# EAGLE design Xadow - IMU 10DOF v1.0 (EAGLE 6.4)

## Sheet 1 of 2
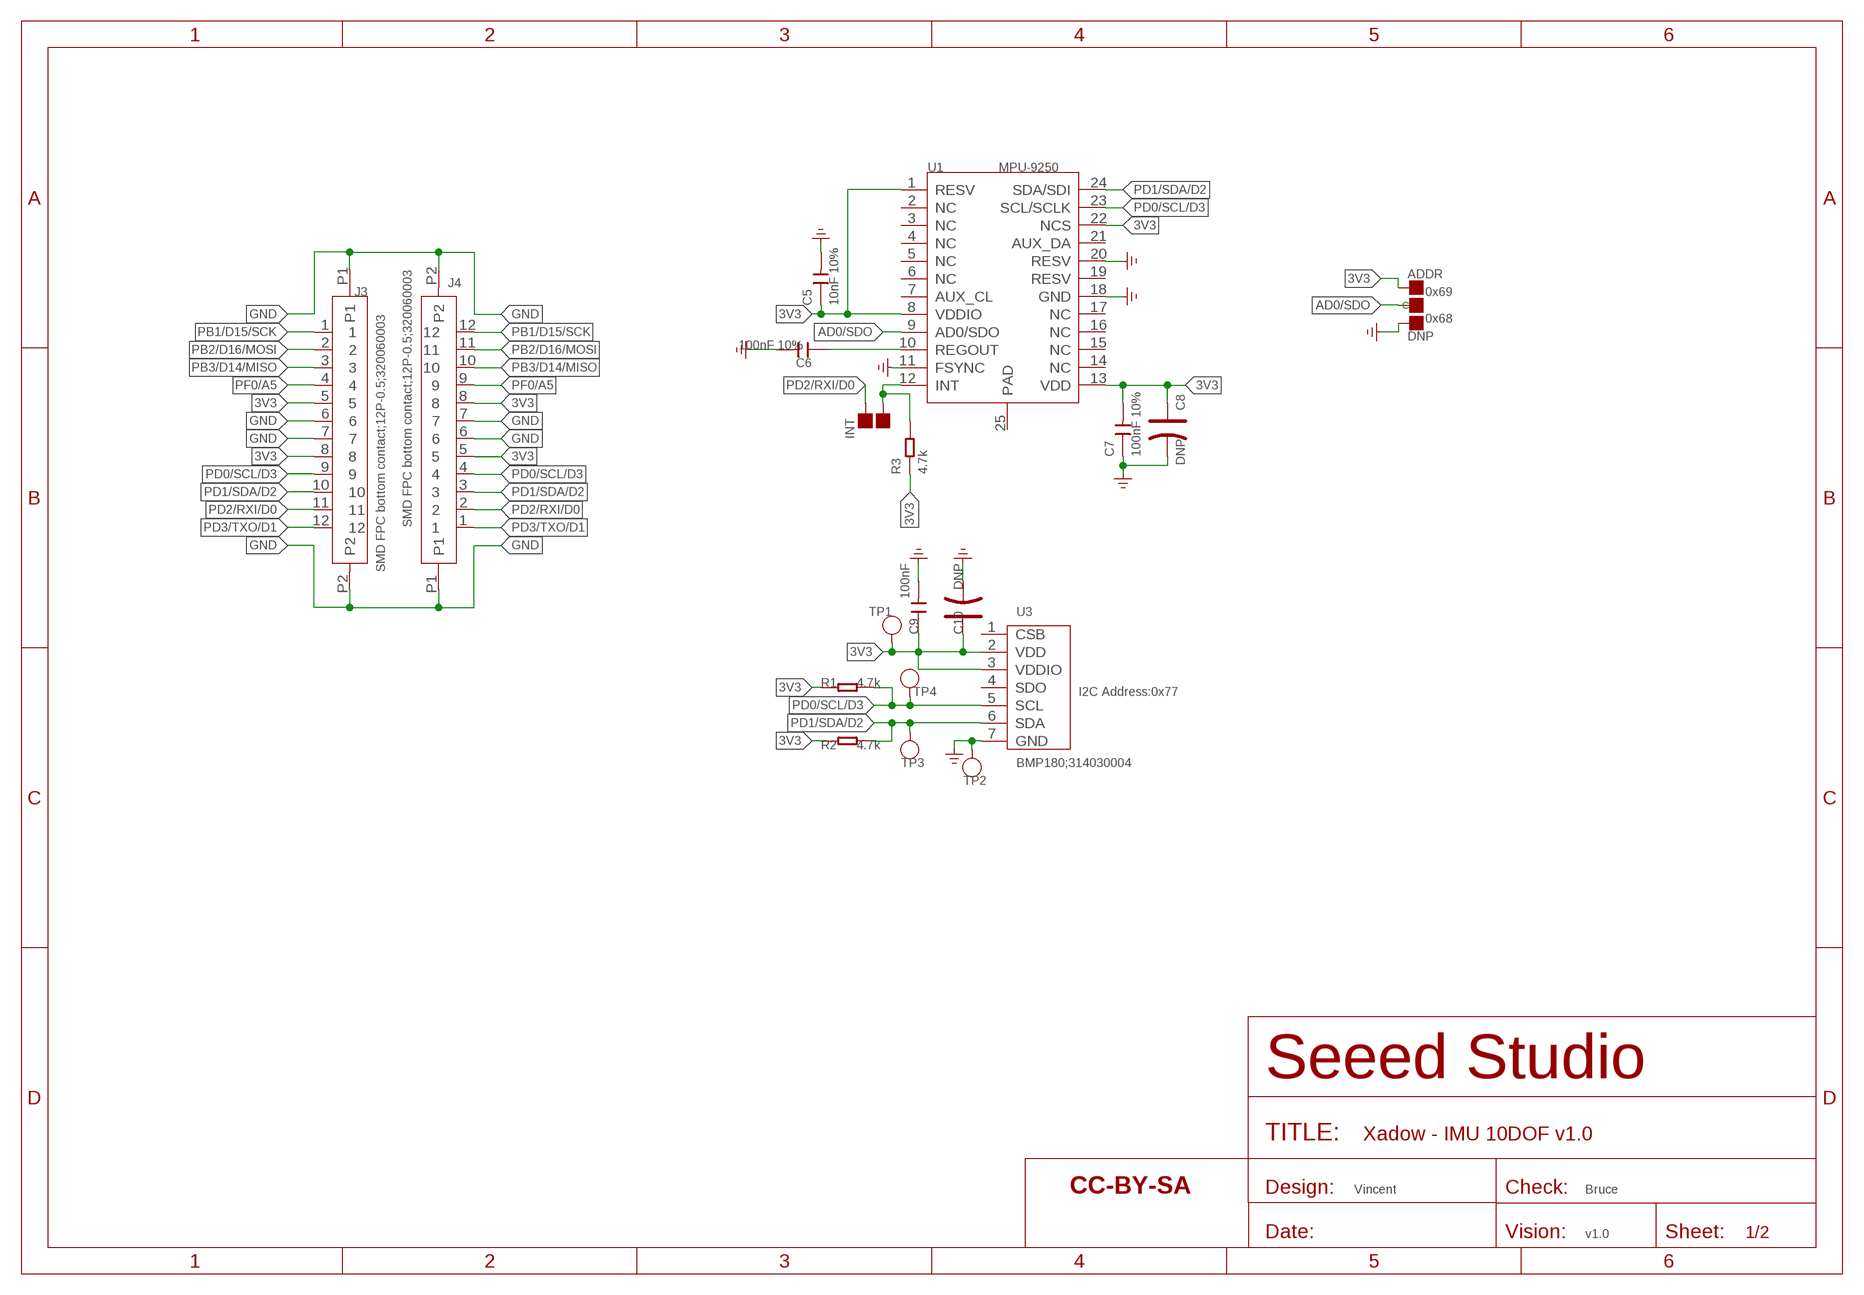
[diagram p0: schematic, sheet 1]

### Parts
ADDR  DNP  PAD-JUMPER-3P-40*40  [3P-SMD-L4.1*W1.5MM]
C5  10nF 10%  CAP-0603  [C0603]
C6  100nF 10%  CAP-0603  [C0603]
C7  100nF 10%  CAP-0603  [C0603]
C8  DNP  CAP-POLAR-AVX-A  [AVX-A]
C9  100nF  CAP-0603  [C0603]
C10  DNP  CAP-POLAR-AVX-A  [AVX-A]
INT  PAD-JUMPER-2P  [2P-SMD-L1.78*W1.27MM]
J3  SMD FPC bottom contact;12P-0.5;320060003  FPC-CONNECTOR-12P-FH12-12S-0.5SH  [12P-0.5]
J4  SMD FPC bottom contact;12P-0.5;320060003  FPC-CONNECTOR-12P-FH12-12S-0.5SH  [12P-0.5]
R1  4.7k  RES-0603  [R0603]
R2  4.7k  RES-0603  [R0603]
R3  4.7k  RES-0603  [R0603]
TP1  PAD-TEST-POINT'4545'  [TP-D45MIL]
TP2  PAD-TEST-POINT'4545'  [TP-D45MIL]
TP3  PAD-TEST-POINT'4545'  [TP-D45MIL]
TP4  PAD-TEST-POINT'4545'  [TP-D45MIL]
U1  MPU-9250  [LEAD-QFN24]
U3  BMP180;314030004  BMP180  [LGA-7]
U$1  SEEEDSTUDIO-OPEN-SCH-FRAME  [SEEEDSTUDIO-PCB-FRAME]

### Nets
3V3: ADDR.00(L) C5.1 C7.2 C8.+ C9.1 C10.+ J3.5 J3.8 J4.5 J4.8 R1.1 R2.1 R3.1 TP1.T U1.1(RESV) U1.8(VDDIO) U1.13(VDD) U1.22(NCS) U3.2(VDD) U3.3(VDDIO)
AD0/SDO: ADDR.MM(C) U1.9(AD0/SDO)
GND: ADDR.11(R) C5.2 C6.2 C7.1 C8.- C9.2 C10.- J3.6 J3.7 J3.P1 J3.P2 J4.6 J4.7 J4.P1 J4.P2 TP2.T U1.11(FSYNC) U1.18(GND) U1.20(RESV) U3.7(GND) ; supply symbol labelled GND_POWER
N$3: C6.1 U1.10(REGOUT)
N$4: INT.1 R3.2 U1.12(INT)
PB1/D15/SCK: J3.1 J4.12
PB2/D16/MOSI: J3.2 J4.11
PB3/D14/MISO: J3.3 J4.10
PD0/SCL/D3: J3.9 J4.4 R1.2 TP4.T U1.23(SCL/SCLK) U3.5(SCL)
PD1/SDA/D2: J3.10 J4.3 R2.2 TP3.T U1.24(SDA/SDI) U3.6(SDA)
PD2/RXI/D0: INT.2 J3.11 J4.2
PD3/TXO/D1: J3.12 J4.1
PF0/A5: J3.4 J4.9
Unconnected: U1.2(NC) U1.3(NC) U1.4(NC) U1.5(NC) U1.6(NC) U1.7(AUX_CL) U1.14(NC) U1.15(NC) U1.16(NC) U1.17(NC) U1.19(RESV) U1.21(AUX_DA) U1.25(PAD) U3.1(CSB) U3.4(SDO)

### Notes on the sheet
- 0x69
- 0x68
- I2C Address:0x77
- Vincent | Bruce
- v1.0

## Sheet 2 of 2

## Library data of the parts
ADDR = Discrete-new:PAD-JUMPER-3P; PARTNO: DNP
C5-C7 C9 = Discrete-new:CAP: Ceramic Capacitors
C8 C10 = Discrete-new:CAP-POLAR: Electrolytic Capacitors,Tantalum Capacitors and Super Capacitors
INT = Discrete-new:PAD-JUMPER-2P; PARTNO: DNP
J3 J4 = Connector-new:FPC-CONNECTOR-12P: 320060003
R1-R3 = Discrete-new:RES
TP1-TP4 = Discrete-new:PAD-TEST-POINT; PARTNO: DNP
U1 = template:MPU-9250
U3 = template:BMP180: Digital pressure sensor
U$1 = moudle-new:SEEEDSTUDIO-OPEN-SCH-FRAME

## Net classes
0 default: width 0.152 mm, drill 0.305 mm, clearance 0.152 mm

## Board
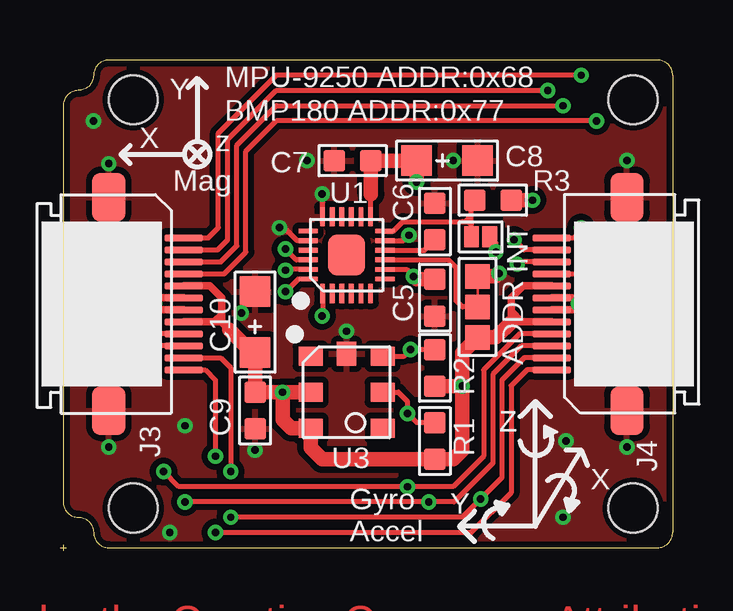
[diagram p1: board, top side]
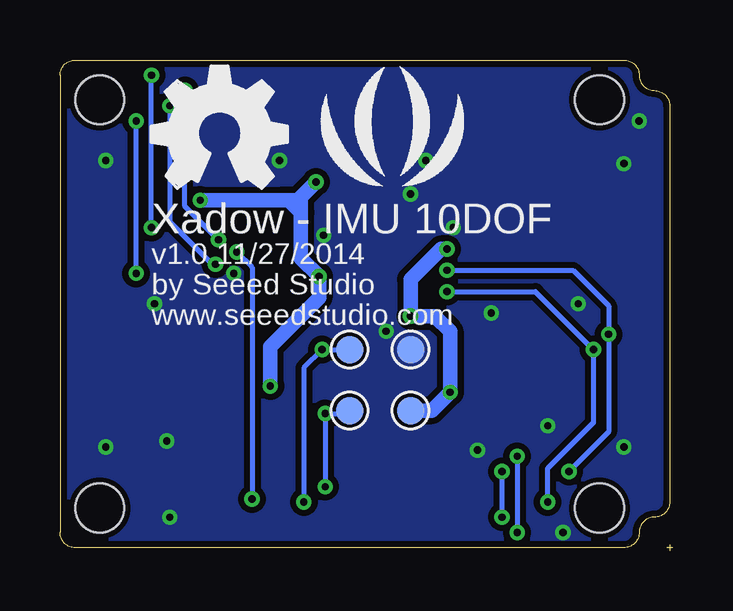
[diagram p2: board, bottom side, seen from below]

Size 25.53 x 20.45 mm. Coordinates in mm from the lower left corner, seen from the top.
Copper layers (1*16): Top 0.035mm / dielectric 1.5mm / Bottom 0.035mm
Design rules "SeeedStudio_2layer_DRU_no_angle_20140221 *": minimum track width 6mil, minimum drill 12mil, track to track 6mil, track to pad 6mil, pad to pad 6mil, via to via 6mil, smd to smd 0mil, copper to edge 10mil, drill to drill 10mil, minimum pad ring 10mil, minimum via ring 6mil, stop-mask expansion 2mil, vias tented up to drill 25mil, thermal gap 10mil

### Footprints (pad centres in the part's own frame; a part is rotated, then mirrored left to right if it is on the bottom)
3P-SMD-L4.1*W1.5MM = smd 1.016 x 1.016: 00 -1.27,0; 11 1.27,0; MM 0,0
C0603 = smd 0.889 x 0.889: 1 0,0.762; 2 0,-0.762
AVX-A = smd 1.27 x 1.27: + -1.27,0; - 1.27,0
2P-SMD-L1.78*W1.27MM = smd 0.889 x 0.61: 1 0,0.381; 2 0,-0.381
12P-0.5 = smd 0.3 x 1.6: 1 -2.75,3.127; 2 -2.25,3.127; 3 -1.75,3.127; 4 -1.25,3.127; 5 -0.75,3.127; 6 -0.25,3.127; 7 0.25,3.127; 8 0.75,3.127; 9 1.25,3.127; 10 1.75,3.127; 11 2.25,3.127; 12 2.75,3.127 | smd 2.032 x 1.397: P1 -4.445,0; P2 4.445,0
R0603 = smd 0.889 x 0.889: 1 0,0.762; 2 0,-0.762
TP-D45MIL = smd 1.143 x 1.143: T 0,0
LEAD-QFN24 = smd 0.8 x 0.2: 1 -1.6,1; 2 -1.6,0.6; 3 -1.6,0.2; 4 -1.6,-0.2; 5 -1.6,-0.6; 6 -1.6,-1; 13 1.6,-1; 14 1.6,-0.6; 15 1.6,-0.2; 16 1.6,0.2; 17 1.6,0.6; 18 1.6,1 | smd 0.2 x 0.8: 7 -1,-1.6; 8 -0.6,-1.6; 9 -0.2,-1.6; 10 0.2,-1.6; 11 0.6,-1.6; 12 1,-1.6; 19 1,1.6; 20 0.6,1.6; 21 0.2,1.6; 22 -0.2,1.6; 23 -0.6,1.6; 24 -1,1.6 | smd 1.7 x 1.54: 25 0,0
LGA-7 = smd 0.8 x 1: 1 1.5,1.5; 2 0,1.5; 3 -1.5,1.5; 4 -1.5,-1.5; 5 0,-1.5; 6 1.5,-1.5 | smd 1 x 0.8: 7 1.6,0
XADOW-DRILL-DIM-25*20MM = hole 2.032: -9.779,-8.509; -9.779,8.509; 11.049,8.509; 11.049,-8.509

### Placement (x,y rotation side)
ADDR  17.4,10.16 90 top
C5  15.62,10.54 0 top
C6  15.62,13.72 180 top
C7  12.19,16.26 90 top
C8  16.13,16.26 0 top
C9  8.13,5.84 0 top
C10  8.13,9.53 90 top
INT  17.53,13.08 90 top
J3  2.03,10.29 270 top
J4  23.62,10.29 90 top
R1  15.62,4.57 180 top
R2  15.62,7.62 180 top
R3  18.03,14.61 270 top
TP1  10.92,5.84 90 bottom
TP2  10.92,8.38 90 bottom
TP3  13.46,8.38 90 bottom
TP4  13.46,5.84 90 bottom
U1  11.94,12.32 90 top
U3  11.94,6.6 90 top
U$1  not placed on the board
U$2  [OSHW_FILLX200_NOTEXT]  21.72,15.11 0 bottom
U$3  [SEEED-SILK-280*268MIL]  11.68,16.89 0 bottom
U$4  [XADOW-DRILL-DIM-25*20MM]  12.83,10.29 0 top
U$15  [XADOW-DRILL-DIM-25*20MM]  12.83,10.29 0 top

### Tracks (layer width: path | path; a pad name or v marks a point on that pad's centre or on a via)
3V3  (via drill 0.3 pad 0.64)
  Top 0.203: U1.13 12.94,14.84 12.95,14.86 | U1.8 14.44,11.72 v14.73,11.43 | U1.1 10.94,9.79 v10.92,9.78 | U1.22 9.85,12.12 v9.4,12.57
  Top 0.305: J3.8 6.72,9.54 | 6.72,9.54 7.05,9.21 7.11,9.14 | J3.5 6.24,11.04 6.73,10.54 6.73,9.84 | 6.73,9.84 6.73,9.55 6.72,9.54 | 6.73,9.84 6.48,9.59 | J4.5 18.81,9.54 18.8,9.53 18.8,9.91 | J4.8 19.29,11.04 18.8,10.54 18.8,9.91 | 18.8,9.91 18.86,9.91 19.18,9.59
  Top 0.61: 12.95,14.86 C7.2 C8.+ v14.86,15.37 | v9.27,6.6 C9.1 C10.+ 8,8.26 7.05,9.21 | U3.2 v9.27,6.6 | v16.76,6.86 16.76,4.19 16.38,3.81 R1.1 10.92,3.81 10.44,4.29 U3.3 9.63,5.1 9.27,5.46 v9.27,6.6 | C5.1 14.86,11.3 v14.73,11.43 | R2.1 v16.76,6.86 | v16.76,6.86 16.76,8.26 ADDR.00 18.16,8.89 18.8,9.53 | R3.1 v19.69,14.61
  Bottom 0.61: TP1.T 10.03,5.84 v9.27,6.6 9.27,9.14 9.91,9.78 v10.92,9.78 10.92,11.3 9.65,12.57 v9.4,12.57 | v16.76,6.86 16.76,8.51 14.73,10.54 v14.73,11.43 15.49,12.19 15.49,14.1 | 15.49,14.1 15.49,14.61 | 15.49,14.61 15.49,14.73 v14.86,15.37 | v19.69,14.61 16.26,14.61 16,14.61 | 16,14.61 15.49,14.61 | 16,14.61 15.49,14.1
AD0/SDO
  Top 0.203: U1.9 16.18,12.12 16.51,11.79 16.51,10.41 16.76,10.16 ADDR.MM
GND  (via drill 0.3 pad 0.64)
  Top 0.102: ADDR.11 17.4,10.16
  Top 0.203: U1.20 9.88,12.92 9.33,13.46 v9.14,13.46 | U1.11 14.32,12.92 v14.54,13.15 | U1.18 10.94,14.84 v10.92,14.86
  Top 0.305: J3.6 4.19,10.54 v3.94,10.29 4.19,10.04 J3.7 | J4.7 21.34,10.54 v21.59,10.29 21.34,10.04 J4.6
  Top 0.61: ADDR.11 18.16,11.43 v18.29,11.56
  other vias: 8.13,4.19 11.94,9.14 7.56,9.91 23.62,4.32 23.62,16.26 2.03,4.32 2.03,16.13 1.4,17.91 21.08,4.57 20.95,1.4 10.29,16.26 16.38,16.26 4.57,0.76 5.21,5.21
  pour Bottom (isolate 0.254, rank 6): -0.51,21.08 26.16,21.08 26.16,-0.51 -0.51,-0.51
  pour Top (isolate 0.254, rank 6): -0.51,21.08 26.16,21.08 26.16,-0.51 -0.51,-0.51
N$3
  Top 0.203: U1.10 15.19,12.52 C6.1
N$4
  Top 0.203: 16.89,13.72 17.15,13.72 | U1.12 13.89,13.32 14.29,13.72 16.76,13.72 16.89,13.72 | INT.1 17.15,13.59 | 17.15,13.59 17.15,13.72 | 17.15,13.72 17.15,13.97 | 17.15,13.97 17.15,14.48 R3.2 | 16.89,13.72 17.15,13.97 | 16.89,13.72 17.02,13.72 17.15,13.59
PB1/D15/SCK  (via drill 0.3 pad 0.64)
  Top 0.203: J3.1 6.18,13.04 6.6,13.46 6.6,17.4 9.02,19.81 v21.72,19.81 | J4.12 21.42,13.04 21.72,13.34 v21.72,13.46
  Bottom 0.203: v21.72,13.46 v21.72,19.81
PB2/D16/MOSI  (via drill 0.3 pad 0.64)
  Top 0.203: J3.2 6.57,12.54 6.99,12.95 6.99,17.15 9.02,19.18 v20.32,19.18 | J4.11 19.34,12.54 v18.92,12.95
  Bottom 0.203: v18.92,12.95 20.32,14.35 v20.32,19.18
PB3/D14/MISO  (via drill 0.3 pad 0.64)
  Top 0.203: J3.3 6.7,12.04 7.37,12.7 7.37,16.89 9.02,18.54 v20.95,18.54 | J4.10 19.15,12.04 v19.05,11.94
  Bottom 0.203: v20.95,18.54 20.95,13.72 20.7,13.46 20.64,13.4 19.18,11.94 v19.05,11.94
PD0/SCL/D3  (via drill 0.3 pad 0.64)
  Top 0.203: U1.23 9.43,11.72 v9.4,11.68 | J3.9 2.69,9.04 v2.67,9.02 | R1.2 14.86,5.33 v14.48,5.72 14.48,6.22 14.1,6.6 U3.5 | J4.4 19.15,9.04 17.65,7.54 17.65,3.94 16.38,2.67 v14.48,2.67 4.95,2.67 v4.32,3.3
  Bottom 0.203: v9.4,11.68 4.15,11.68 2.67,10.2 v2.67,9.02 2.67,4.95 v4.32,3.3 | TP4.T 13.59,5.72 v14.48,5.72 v14.48,2.67
PD1/SDA/D2  (via drill 0.3 pad 0.64)
  Top 0.203: J3.10 3.46,8.54 v3.3,8.38 | U1.24 9.92,11.32 v9.4,10.79 | U3.6 14.33,8.1 v14.61,8.38 R2.2 | J4.3 19.23,8.54 18.03,7.35 18.03,3.65 16.42,2.03 v15.37,2.03 v5.21,2.03
  Bottom 0.203: v9.4,10.79 5.72,10.79 v3.3,8.38 3.3,5.33 5.21,3.43 v5.21,2.03 | TP3.T v14.61,8.38 15.37,7.62 v15.37,2.03
PD2/RXI/D0  (via drill 0.3 pad 0.64)
  Top 0.203: J4.2 19.34,8.04 18.41,7.11 18.41,3.05 v17.53,2.16 16.76,1.4 v7.11,1.4 | J3.11 6.7,8.04 7.11,7.62 v7.11,3.3 | v18.16,12.45 18.16,12.83 INT.2
  Bottom 0.203: v7.11,3.3 v7.11,1.4 | v17.53,2.16 17.53,11.81 v18.16,12.45
PD3/TXO/D1  (via drill 0.3 pad 0.64)
  Top 0.203: J3.12 6.05,7.54 6.48,7.11 v6.48,3.94 | v6.48,0.76 17.15,0.76 18.8,2.41 18.8,6.88 19.46,7.54 J4.1
  Bottom 0.203: v6.48,3.94 v6.48,0.76
PF0/A5  (via drill 0.3 pad 0.64)
  Top 0.203: J3.4 6.84,11.54 7.75,12.45 7.75,16.64 9.02,17.91 v22.35,17.91 | J4.9 22.33,11.54 v22.35,11.56
  Bottom 0.203: v22.35,11.56 v22.35,17.91

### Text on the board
tPlace: Y | MPU-9250 ADDR:0x68 | BMP180 ADDR:0x77 | X | z | Mag | Z | X | Y | Gyro / Accel
bPlace: Xadow - IMU 10DOF | v1.0 11/27/2014 | by Seeed Studio | www.seeedstudio.com
Patch_Top: Top Enhance 0.25~0.28mm
Vscore: Bottom Enhance
tMap: Holes on Bottom Enhance | All Holes are 70mil diameter

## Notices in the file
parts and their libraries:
moudle-new: This work is licensed under the Creative Commons Attribution 4.0 International License.
To view a copy of this license,visit:
http://creativecommons.org/licenses/by-sa/4.0
moudle-new: CC-BY-SA
